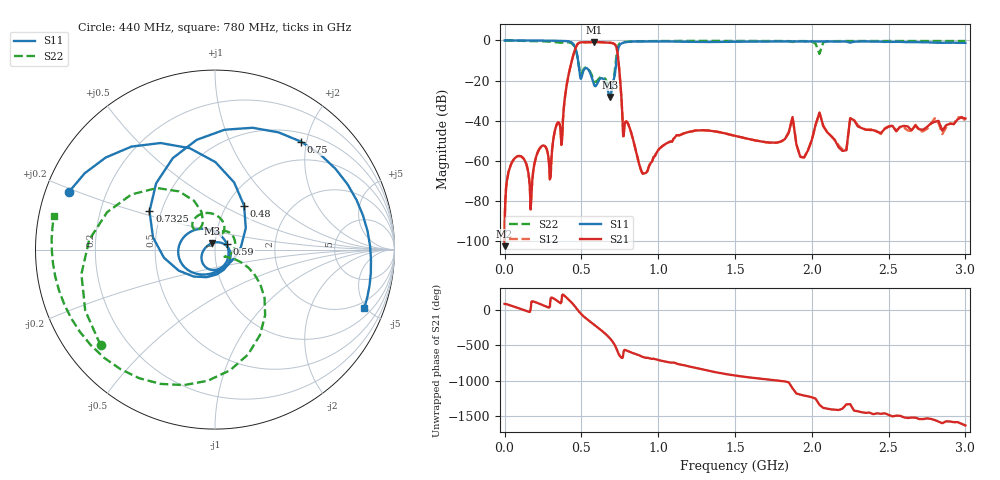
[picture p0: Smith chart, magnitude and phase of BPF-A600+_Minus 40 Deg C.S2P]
! Mini-Circuits
! S2P DATA File Format
! Type: BAND PASS FILTER
! Model:BPF-A600+
! All S Parameters are in dB deg format
! TEST CONDITIONS: INPUT POWER = 0 dBm @ Temperature = - 40 deg C
! 401 Frequency points
# MHz S DB R 50
!FREQMAG(S11)PHS(S11)MAG(S21)PHS(S21)MAG(S12)PHS(S12)MAG(S22)PHS(S22)
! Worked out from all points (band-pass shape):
!   401 points, 500 kHz to 3 GHz, reference 50 ohm
!   highest |S21| = -0.76 dB at 585 MHz (marker M1); lowest = -102.5 dB at 500 kHz (marker M2)
!   |S21| within 3 dB of the highest: 462.5 MHz to 729.3 MHz (266.8 MHz wide, 44.8 % of centre)
!   lowest |S11| = -28.1 dB at 685 MHz (marker M3), VSWR 1.08, Z = 48.4 + j3.51 ohm
!   |S11| at or under -10 dB: 478.7 MHz to 728.7 MHz (250 MHz wide, 41.4 % of centre)
!   |S22| runs from -23.6 to 0.0 dB; largest |S21 - S12| = 0.0023
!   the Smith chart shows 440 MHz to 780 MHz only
!   S11 on the Smith chart (normalised r, x): 440 MHz: 0.07, +0.19; 480 MHz: 1.20, +0.64; 590 MHz: 1.14, +0.07; 732.5 MHz: 0.43, +0.22; 750 MHz: 0.65, +1.90; 780 MHz: 1.48, -4.82
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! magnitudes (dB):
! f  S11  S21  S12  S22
! 500 kHz  0.0  -102.5  -100.2  0.0
! 75 MHz  0.0  -58.1  -58.1  -0.1
! 170 MHz  0.0  -84.2  -83.3  -0.3
! 235 MHz  0.0  -53.2  -53.2  -0.4
! 300 MHz  -0.1  -68.2  -68.0  -0.5
! 335 MHz  -0.1  -42.9  -42.9  -0.9
! 375 MHz  -0.2  -49.1  -49.1  -1.1
! 440 MHz  -1.2  -9.5  -9.5  -1.6
! 480 MHz  -10.6  -1.5  -1.5  -10.6
! 502.5 MHz  -18.0  -0.9  -0.9  -16.3
! 585 MHz  -22.4  -0.8  -0.8  -20.2
! 590 MHz  -22.8  -0.8  -0.8  -20.5
! 685 MHz  -28.1  -1.1  -1.1  -23.2
! 732.5 MHz  -7.5  -4.9  -4.9  -5.4
! 750 MHz  -2.3  -17.3  -17.3  -1.4
! 780 MHz  -1.0  -43.0  -43.0  -0.8
! 897.5 MHz  -0.4  -65.8  -66.2  -0.4
! 1.01 GHz  -0.4  -53.8  -53.8  -0.3
! 1.51 GHz  -0.6  -47.6  -47.7  -0.2
! 2.025 GHz  -0.5  -42.0  -42.0  -1.6
! 2.525 GHz  -0.7  -42.5  -42.4  -0.3
! 3 GHz  -1.2  -38.9  -39.9  -0.3
